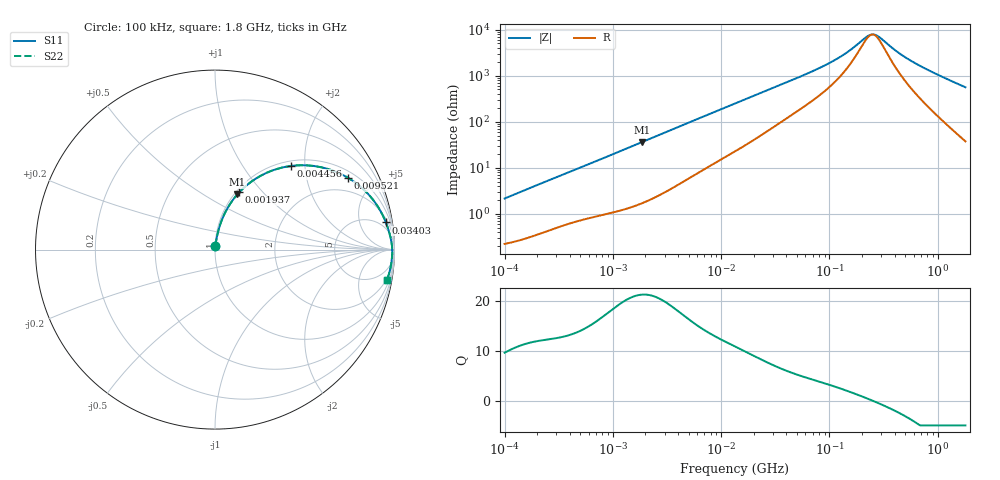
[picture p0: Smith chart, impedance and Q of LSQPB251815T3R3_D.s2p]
! LSQPB251815T3R3_D  S-PARAMETER MODEL  ( General Type )
! Model Generated by TAIYO YUDEN Corporation (http://www.ty-top.com)
! Version 2.0
! TAIYO YUDEN Control No. 110926NG22SB-FKC
! Copyright(c) 2010 TAIYO YUDEN CO.,LTD. All Rights Reserved.
! Product Description (link to TY-COMPAS)
! https://ds.yuden.co.jp/TYCOMPAS/or/detail?pn=LSQPB251815T3R3MD&u=M
! Products Name : Inductors
! Characteristics :
!  Inductance : 3.3 uH , SRF(min) : 200 MHz , DC Resistance(max) : 0.2145 Ohm
!  Rated Current : Saturation :1200 mA , Temp Rise : 800 mA (40 degC)
!  Case Size : 2.5 x 1.8 / 0.098 x 0.071 [mm/inch] , Thickness : 1.5 / 0.06 [mm/inch]
!  (Conditions: Temperature = 25 degC , DC Bias Current/Voltage = 0A / 0V)
! External Node Assignments :
!  1  o---GGG---o  2
! GND o---------o GND
! Frequency Range : 0.1MHz  -  1800MHz  [ 402 STEP ]
# MHz S RI R 50
! Freq[MHz].  S11 Real  S11 Imag  S21 Real  S21 Imag  S12 Real  S12 Imag  S22 Real  S22 Imag
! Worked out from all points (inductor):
!   401 points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, 100 kHz to 1.8 GHz, reference 50 ohm
!   read as one part in series: L = 3.37 uH near 105 kHz
!   highest Q = 21.3 at 1.845 MHz (marker M1), where L = 3.08 uH
!   self-resonance near 249.1 MHz
!   S11 on the Smith chart (normalised r, x): 100 kHz: 1.00, +0.04; 1.937 MHz: 1.04, +0.75; 4.456 MHz: 1.10, +1.70; 9.521 MHz: 1.28, +3.53; 34.03 MHz: 3, +12; 1.8 GHz: 2, -11
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0.1  0.00265 0.0212  0.9973 -0.0212  0.9973 -0.0212  0.00265 0.0212
0.516129  0.0176 0.1008  0.9824 -0.1008  0.9824 -0.1008  0.0176 0.1008
1.076226  0.052 0.1972  0.948 -0.1972  0.948 -0.1972  0.052 0.1972
1.844776  0.1246 0.3077  0.8754 -0.3077  0.8754 -0.3077  0.1246 0.3077
1.937403  0.1348 0.3189  0.8652 -0.3189  0.8652 -0.3189  0.1348 0.3189
2.66389  0.2199 0.3906  0.7801 -0.3906  0.7801 -0.3906  0.2199 0.3906
4.455722  0.4241 0.466  0.5759 -0.466  0.5759 -0.466  0.4241 0.466
6.278453  0.5793 0.4611  0.4207 -0.4611  0.4207 -0.4611  0.5793 0.4611
9.52142  0.742 0.3994  0.258 -0.3994  0.258 -0.3994  0.742 0.3994
13.41641  0.8374 0.326  0.1626 -0.326  0.1626 -0.326  0.8374 0.326
20.3463  0.9086 0.2376  0.0914 -0.2376  0.0914 -0.2376  0.9086 0.2376
34.03197  0.952 0.1513  0.048 -0.1513  0.048 -0.1513  0.952 0.1513
69.24595  0.976 0.0755  0.024 -0.0755  0.024 -0.0755  0.976 0.0755
127.7465  0.9843 0.0342  0.0157 -0.0342  0.0157 -0.0342  0.9843 0.0342
235.6695  0.9873 0.0027  0.0127 -0.0027  0.0127 -0.0027  0.9873 0.0027
253.6402  0.9874 -0.000881  0.0126 0.000881  0.0126 0.000881  0.9874 -0.000881
272.9811  0.9875 -0.00448  0.0125 0.00448  0.0125 0.00448  0.9875 -0.00448
357.3983  0.9875 -0.0181  0.0125 0.0181  0.0125 0.0181  0.9875 -0.0181
467.921  0.9869 -0.033  0.0131 0.033  0.0131 0.033  0.9869 -0.033
659.3364  0.985 -0.0556  0.015 0.0556  0.015 0.0556  0.985 -0.0556
1076.145  0.978 -0.0995  0.022 0.0995  0.022 0.0995  0.978 -0.0995
1800  0.9583 -0.1691  0.0417 0.1691  0.0417 0.1691  0.9583 -0.1691
